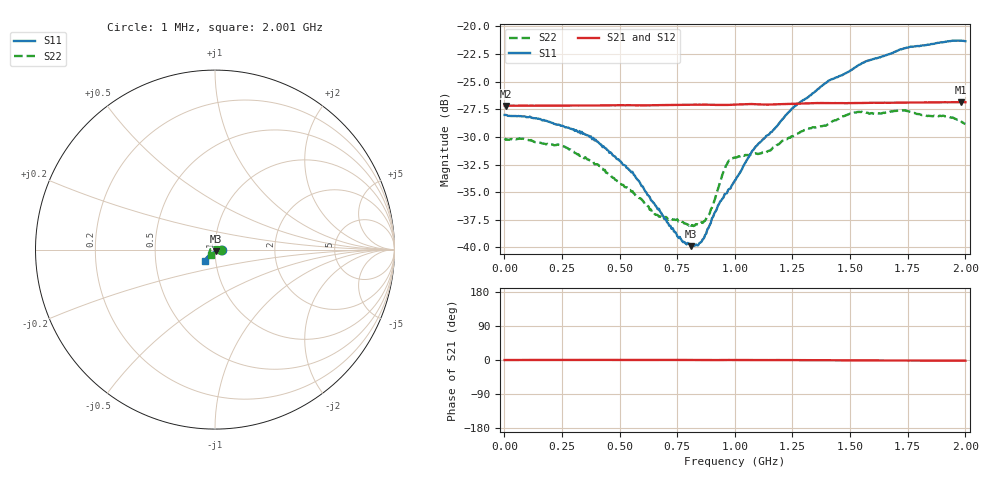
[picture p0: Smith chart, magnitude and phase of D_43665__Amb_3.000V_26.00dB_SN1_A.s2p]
! device id: 43665_
! dir: \\malibu\benchdata\1_engineers\tn_data\43665_75ohm\new\sparar\43665_\amb\3p000v\26p00db
! Serial: 1
! Insertion: A
! Temp: Amb
! VDD: 3.000V
! Attenuation Step: 26.00dB
! IDD: 1.446605e+00mA
! FILE NAME
! DATE 03-27-2009 08:39:45
! CORRECTED  DATA
#  Hz  S  RI  R  75
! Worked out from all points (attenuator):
!   401 points, 1 MHz to 2.001 GHz, reference 75 ohm
!   highest |S21| = -26.85 dB at 1.981 GHz (marker M1); lowest = -27.2 dB at 6 MHz (marker M2)
!   lowest |S11| = -39.9 dB at 811 MHz (marker M3), VSWR 1.02, Z = 75.6 - j1.42 ohm
!   |S11| at or under -10 dB: start of sweep to end of sweep
!   |S22| runs from -38.1 to -27.6 dB; largest |S21 - S12| = 0.00027
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1000000  0.0398 -0.00026  0.0438 -3.58e-05  0.0439 5.94e-05  0.0312 -0.000154
6000000  0.0397 -0.000452  0.0436 -2.75e-05  0.0438 1.85e-05  0.0307 0.00024
2.41e8  0.0357 -0.000552  0.0438 9.63e-05  0.0438 0.000181  0.0269 0.0109
3.36e8  0.0333 -0.00105  0.0438 0.000132  0.0439 0.000179  0.0218 0.0141
3.96e8  0.0307 -0.000922  0.0439 0.000195  0.0439 0.000229  0.0185 0.015
5.46e8  0.0221 -0.00289  0.044 0.000109  0.044 0.000196  0.00929 0.0156
6.71e8  0.0138 -0.00578  0.044 0.000153  0.0441 0.000251  0.000948 0.0137
7.61e8  0.00765 -0.00811  0.0441 0.000106  0.0442 0.000216  -0.00538 0.0119
8.11e8  0.00381 -0.00938  0.0442 7.69e-05  0.0442 0.000172  -0.00878 0.00894
8.46e8  0.0012 -0.0104  0.0442 -2.12e-05  0.0442 9.66e-05  -0.0109 0.00672
8.81e8  -0.00186 -0.0119  0.0442 -6.68e-05  0.0443 4.19e-05  -0.0132 0.00396
9.61e8  -0.00809 -0.0155  0.0441 -2.03e-05  0.0441 0.000118  -0.0233 0.00077
1.001e9  -0.0115 -0.0165  0.0443 8.58e-05  0.0443 0.000195  -0.0254 0.00207
1.096e9  -0.0197 -0.0211  0.0444 -0.000344  0.0445 -0.000174  -0.0264 -0.00247
1.146e9  -0.0226 -0.0231  0.0443 -0.000207  0.0444 -3.44e-05  -0.0269 -0.0051
1.251e9  -0.031 -0.0293  0.0446 -0.000168  0.0447 3.48e-06  -0.0295 -0.0118
1.336e9  -0.0363 -0.0338  0.0449 -0.00038  0.0451 -0.000173  -0.0311 -0.0159
1.531e9  -0.0478 -0.0456  0.045 -0.000822  0.0452 -0.000672  -0.0321 -0.0255
1.671e9  -0.0527 -0.0534  0.0452 -0.000999  0.0453 -0.000889  -0.0299 -0.0279
1.736e9  -0.0545 -0.0581  0.0452 -0.00111  0.0454 -0.00101  -0.0287 -0.0302
1.981e9  -0.0558 -0.0657  0.0454 -0.00137  0.0455 -0.00134  -0.0229 -0.0295
2.001e9  -0.0552 -0.0656  0.0454 -0.00138  0.0455 -0.00139  -0.0223 -0.0284
